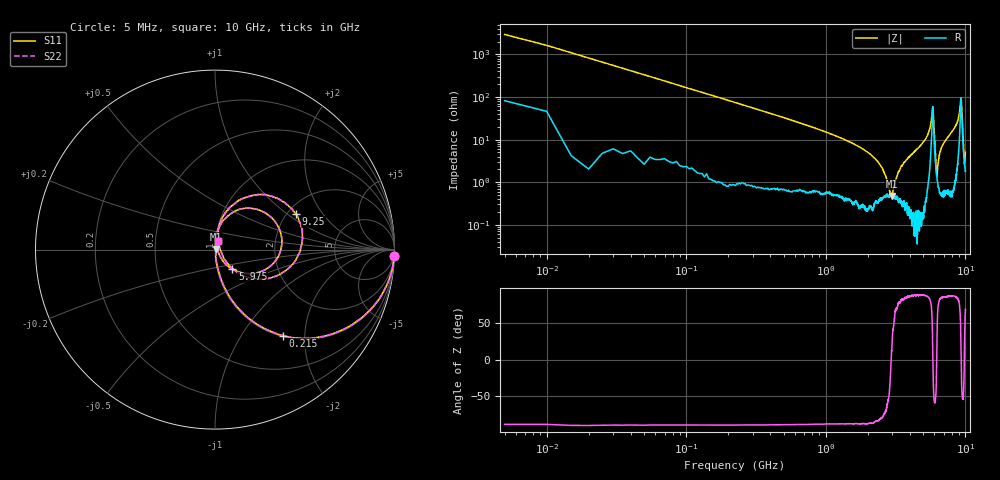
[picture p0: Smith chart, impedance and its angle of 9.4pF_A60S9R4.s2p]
! Amotech Co.,Ltd.
! http://www.amotech.co.kr/
! Part Number: A60S9R4
! These Parameters are Measured in Series Mode Connection
! Operation Temp=25[degC], DC Bias Voltage=0[V]
! Freq. Start=5[MHz] Stop=10[GHz], 2000[Steps]
! Date: Monday, July 13, 2020, 01:34:57
# GHZ S RI R 50.000000
!Freq.(Hz) S11(Real) S11(Imag) S21(Real) S21(Imag) S12(Real) S12(Imag) S22(Real) S22(Imag)
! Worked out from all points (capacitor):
!   2000 points, 5 MHz to 10 GHz, reference 50 ohm
!   read as one part in series: C = 9.55 pF near 55 MHz
!   lowest |Z| = 478 mohm at 2.98 GHz (marker M1)
!   series resonance near 2.939 GHz, so ESL is about 310 pH
!   S11 on the Smith chart (normalised r, x): 5 MHz: 3, -59; 215 MHz: 1.02, -1.55; 5.975 GHz: 1.18, -0.26; 9.25 GHz: 2.23, +1.17; 10 GHz: 1.04, +0.09
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0.005  0.9979 -0.0339  0.0021 0.0339  0.0021 0.0339  0.9979 -0.0339
0.085  0.7893 -0.4  0.2107 0.4  0.2107 0.4  0.7893 -0.4
0.215  0.3777 -0.4792  0.6223 0.4792  0.6223 0.4792  0.3777 -0.4792
0.57  0.0802 -0.2614  0.9198 0.2614  0.9198 0.2614  0.0802 -0.2614
1.675  0.00853 -0.0714  0.9915 0.0714  0.9915 0.0714  0.00853 -0.0714
2.415  0.0046 -0.0268  0.9954 0.0268  0.9954 0.0268  0.0046 -0.0268
2.98  0.00437 0.00187  0.9956 -0.00187  0.9956 -0.00187  0.00437 0.00187
3.34  0.00403 0.0177  0.996 -0.0177  0.996 -0.0177  0.00403 0.0177
5.005  0.00908 0.0872  0.9909 -0.0872  0.9909 -0.0872  0.00908 0.0872
5.6  0.0636 0.1798  0.9364 -0.1798  0.9364 -0.1798  0.0636 0.1798
5.815  0.3521 0.1286  0.6479 -0.1286  0.6479 -0.1286  0.3521 0.1286
5.895  0.2581 -0.1215  0.7419 0.1215  0.7419 0.1215  0.2581 -0.1215
5.975  0.0972 -0.1092  0.9028 0.1092  0.9028 0.1092  0.0972 -0.1092
6.24  0.0132 0.00199  0.9868 -0.00199  0.9868 -0.00199  0.0132 0.00199
6.465  0.00853 0.038  0.9915 -0.038  0.9915 -0.038  0.00853 0.038
6.67  0.00882 0.0574  0.9912 -0.0574  0.9912 -0.0574  0.00882 0.0574
8.335  0.0407 0.1774  0.9593 -0.1774  0.9593 -0.1774  0.0407 0.1774
8.945  0.136 0.2767  0.864 -0.2767  0.864 -0.2767  0.136 0.2767
9.25  0.4516 0.1982  0.5484 -0.1982  0.5484 -0.1982  0.4516 0.1982
9.435  0.2828 -0.1625  0.7172 0.1625  0.7172 0.1625  0.2828 -0.1625
9.825  0.0286 -4.12e-05  0.9714 4.12e-05  0.9714 4.12e-05  0.0286 -4.12e-05
10  0.0195 0.0453  0.9805 -0.0453  0.9805 -0.0453  0.0195 0.0453
